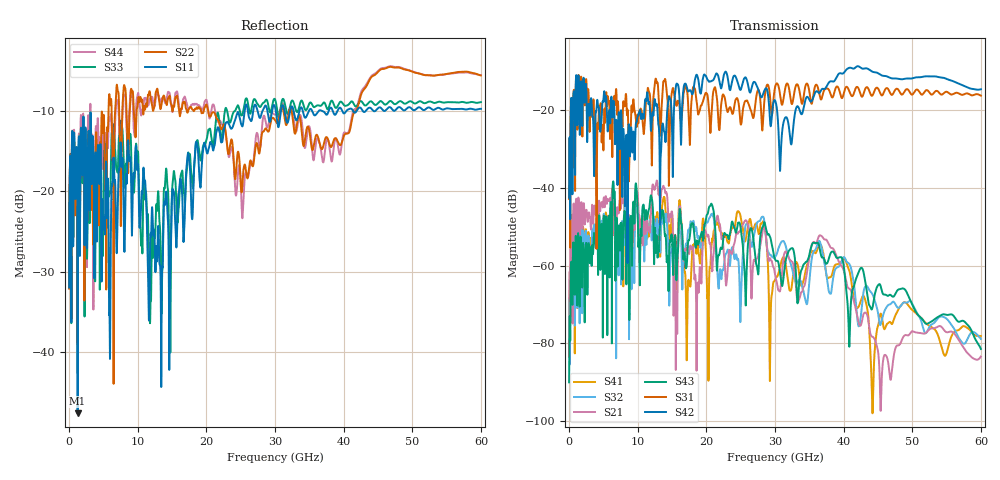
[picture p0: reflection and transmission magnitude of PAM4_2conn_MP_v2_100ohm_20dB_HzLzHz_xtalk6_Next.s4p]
! Info: Touchstone file created by Circ.  Input file=FAB50GbE_2conn_Midplane_Examax_Topo2_v2_100ohm_20dB_HzLzHz.circ
# Hz S RI R 50
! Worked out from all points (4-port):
!   6000 points, 10 MHz to 60 GHz, reference 50 ohm
!   strongest paths, dB at 10 MHz, 15.01 GHz, 30.01 GHz, 45.01 GHz, 60 GHz:
!     S42: -42.5, -25.2, -17.5, -10.5, -14.7
!     S31: -42.9, -15.2, -14.1, -14.4, -16.3
!     S43: -90.0, -52.6, -58.3, -65.0, -81.4
!     S21: -78.3, -46.3, -62.3, -82.0, -83.4
!     S32: -78.8, -54.8, -57.7, -72.1, -78.8
!     S41: -83.4, -46.7, -63.6, -75.4, -78.1
!   lowest |S11| = -47.6 dB at 1.25 GHz (marker M1), VSWR 1.01, Z = 50.4 + j0.0225 ohm
!   |S11| at or under -10 dB: start of sweep to 25.58 GHz; 35.43 GHz to 36.33 GHz (895.3 MHz wide, 2.5 % of centre); 36.89 GHz to 37.81 GHz (926.2 MHz wide, 2.48 % of centre)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
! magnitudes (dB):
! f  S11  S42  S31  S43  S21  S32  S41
! 10 MHz  -32.0  -42.5  -42.9  -90.0  -78.3  -78.8  -83.4
! 1.25 GHz  -47.6  -17.3  -20.0  -54.9  -49.2  -51.6  -51.3
! 8.3 GHz  -17.9  -27.3  -15.9  -55.3  -41.7  -44.5  -50.2
! 20.68 GHz  -14.0  -12.6  -23.4  -44.2  -56.4  -46.9  -56.9
! 30.8 GHz  -10.3  -33.6  -16.7  -62.6  -66.0  -54.3  -60.1
! 36.68 GHz  -9.9  -15.0  -17.3  -57.1  -52.3  -54.6  -54.7
! 60 GHz  -9.7  -14.7  -16.3  -81.4  -83.4  -78.8  -78.1
